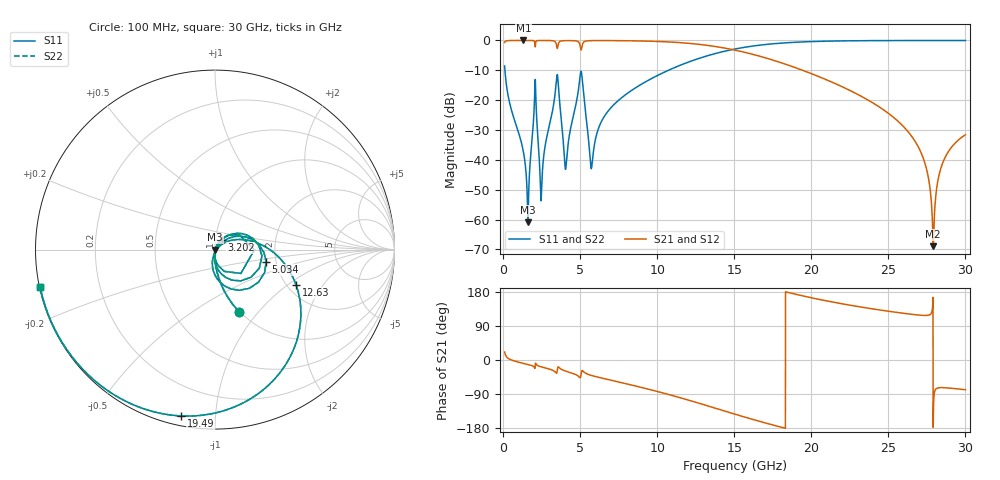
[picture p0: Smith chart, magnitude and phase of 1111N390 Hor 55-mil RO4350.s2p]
# GHz S MA R 50
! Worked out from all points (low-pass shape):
!   3201 points, 100 MHz to 30 GHz, reference 50 ohm
!   highest |S21| = -0.01 dB at 1.324 GHz (marker M1); lowest = -68.9 dB at 27.92 GHz (marker M2)
!   |S21| within 3 dB of the highest: start of sweep to 5.05 GHz; 5.082 GHz to 14.83 GHz (9.748 GHz wide, 97.9 % of centre)
!   lowest |S11| = -60.9 dB at 1.614 GHz (marker M3), VSWR 1.00, Z = 50.1 - j0.0221 ohm
!   |S11| at or under -10 dB: 120.6 MHz to 10.73 GHz (10.61 GHz wide, 196 % of centre)
!   |S22| runs from -60.9 to 0.0 dB; largest |S21 - S12| = 0
!   S11 on the Smith chart (normalised r, x): 100 MHz: 0.99, -0.80; 3.202 GHz: 1.07, +0.11; 5.034 GHz: 1.77, -0.26; 12.63 GHz: 2.23, -1.16; 19.49 GHz: 0.05, -0.82; 30 GHz: 0.00, -0.11
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0.1  0.3731 -68.8  0.9275 21.2  0.9275 21.2  0.3731 -68.8
1.324031  0.01344 -96.1  0.9991 -8.9  0.9991 -8.9  0.01344 -96.1
1.613687  0.0008968 -14.2  0.9989 -11.7  0.9989 -11.7  0.0008968 -14.2
2.0435  0.1089 47.3  0.9538 -20.7  0.9538 -20.7  0.1089 47.3
2.492  0.002946 29.7  0.9977 -18.2  0.9977 -18.2  0.002946 29.7
3.202125  0.06467 55.9  0.9894 -26.8  0.9894 -26.8  0.06467 55.9
3.547844  0.2405 -44.2  0.7755 -19.9  0.7755 -19.9  0.2405 -44.2
4.089781  0.008135 7.8  0.9931 -29.7  0.9931 -29.7  0.008135 7.8
5.0335  0.2931 -13.3  0.7374 -44.7  0.7374 -44.7  0.2931 -13.3
5.089563  0.2884 -48.4  0.7201 -31.4  0.7201 -31.4  0.2884 -48.4
5.743625  0.007338 -18.6  0.9926 -40.9  0.9926 -40.9  0.007338 -18.6
6.818156  0.06578 35.7  0.994 -51.6  0.994 -51.6  0.06578 35.7
10.06978  0.2629 5.6  0.9606 -83.7  0.9606 -83.7  0.2629 5.6
12.62997  0.4923 -23.5  0.865 -113.0  0.865 -113.0  0.4923 -23.5
15.05  0.7186 -53.4  0.6884 -143.0  0.6884 -143.0  0.7186 -53.4
19.48828  0.9458 -101.5  0.3128 168.8  0.3128 168.8  0.9458 -101.5
20.03956  0.9573 -106.4  0.2759 163.9  0.2759 163.9  0.9573 -106.4
25.01978  0.9951 -142.1  0.05973 128.6  0.05973 128.6  0.9951 -142.1
27.12213  0.9969 -153.8  0.01323 118.1  0.01323 118.1  0.9969 -153.8
27.91634  0.997 -157.9  0.0003591 -155.4  0.0003591 -155.4  0.997 -157.9
28.54237  0.9969 -161.0  0.009103 -73.0  0.009103 -73.0  0.9969 -161.0
30  0.9966 -168.0  0.02633 -78.4  0.02633 -78.4  0.9966 -168.0
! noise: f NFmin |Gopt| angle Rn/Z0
0.1  0.0006605  0.7335  1.851  0.0004945
3.417  0.06425  0.8986  24.6  0.1323
6.743  0.02015  0.5101  46.52  0.006152
10.06  0.02486  0.4568  63.25  0.00586
13.39  0.03596  0.5192  78.4  0.00838
16.7  0.05663  0.6377  94.97  0.01424
20.03  0.1025  0.7778  113.9  0.0291
23.35  0.2366  0.8973  133.4  0.07996
26.67  1.202  0.9786  151.6  0.7799
30  1.01  0.9738  167.8  0.1007
